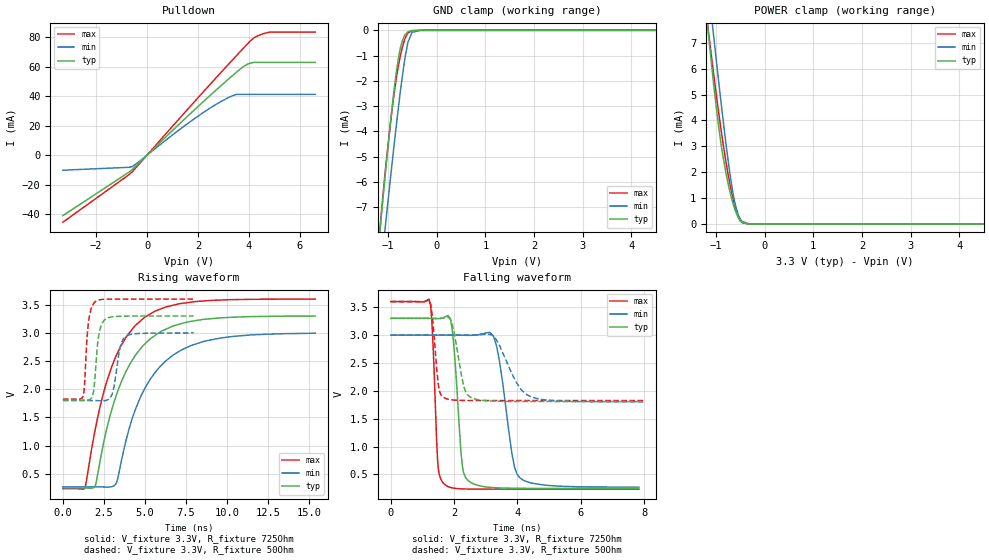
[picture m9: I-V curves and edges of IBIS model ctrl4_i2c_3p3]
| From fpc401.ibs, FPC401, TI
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|   ctrl4_i2c_3p3 Model
[Model]   ctrl4_i2c_3p3
Model_type   I/O_open_drain
Polarity   Non-Inverting
Vinl = 0.8
Vinh = 2
Vmeas = 1.65
Vref = 3.3
Cref = 50pF
Rref = 725
|   typ   min   max
|   (nom PVT)   (fast PVT)   (slow PVT)
C_comp   1.313e-14   1.211e-14   2.018e-14
| Where nom  PVT is Nominal Process, 3.3V, 27C
|   Fast PVT is Strong Process,  3.6V, -40C
|   Slow PVT is Weak Process,   3V, 125C
[Voltage Range]   3.3   3   3.6
|Junction Temperature
[Temperature Range]   27   125   -40
[Pullup Reference]   3.3   3   3.6
[Pulldown Reference]   0   0   0
[Power Clamp Reference]   3.3   3   3.6
[GND Clamp Reference]   0   0   0
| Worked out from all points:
|   slope of the pulldown table from 0 to 0.495 V, typ, clamps not added: 59.6 ohm
|   GND clamp passes 1 mA (typ) near -0.77 V on its own axis
|   POWER clamp passes 1 mA (typ) near -0.68 V on its own axis
|   falling waveform, V_fixture 3.3V, R_fixture 725Ohm: 20-80 % time 216ps typ, 392ps min, 138ps max; typ from 3.3 V to 0.25 V
|   rising waveform, V_fixture 3.3V, R_fixture 725Ohm: 20-80 % time 2.3ns typ, 2.46ns min, 2.13ns max; typ from 0.25 V to 3.3 V
|   falling waveform, V_fixture 3.3V, R_fixture 50Ohm: 20-80 % time 281ps typ, 620ps min, 162ps max; typ from 3.3 V to 1.81 V
|   rising waveform, V_fixture 3.3V, R_fixture 50Ohm: 20-80 % time 290ps typ, 393ps min, 250ps max; typ from 1.81 V to 3.3 V
[Pulldown]
|   Voltage   I(typ)   I(min)   I(max)
-3.3V     -40.84mA   -10.13mA   -45.3mA
-582mV    -9.69mA    -7.733mA   -11.26mA
1.419V    23.6mA     19.21mA    27.73mA
2.042V    33.65mA    26.95mA    39.73mA
2.745V    44.68mA    34.79mA    53.09mA
3.465V    55.55mA    40.96mA    66.6mA
3.792V    60.17mA    41.21mA    72.65mA
3.942V    61.63mA    41.21mA    75.42mA
4.188V    62.83mA    41.21mA    79.35mA
4.469V    62.84mA    41.21mA    81.7mA
4.812V    62.84mA    41.21mA    83.33mA
6.6V      62.84mA    41.21mA    83.34mA
[GND Clamp]
|   Voltage   I(typ)   I(min)   I(max)
-3.3V     -54.89mA   -51.39mA   -65.13mA
-1.185V   -8.379mA   -10.2mA    -8.358mA
-1.136V   -7.374mA   -9.294mA   -7.262mA
-1.063V   -5.874mA   -7.93mA    -5.729mA
-1.036V   -5.337mA   -7.435mA   -5.211mA
-921mV    -3.166mA   -5.372mA   -3.232mA
-813mV    -1.447mA   -3.515mA   -1.711mA
-708mV    -433.5uA   -1.87mA    -696.7uA
-587.4mV  -56.44uA   -464.8uA   -107.3uA
-504mV    -9.281uA   -78.14uA   -15.26uA
-330mV    -89.63nA   -774.9nA   -56.52nA
6.6V      0A         0A         0A
[POWER Clamp]
|   Voltage   I(typ)   I(min)   I(max)
-3.3V     51.03mA    49.04mA    56.86mA
-1.215V   8.494mA    10.26mA    8.507mA
-1.154V   7.358mA    9.183mA    7.481mA
-1.049V   5.476mA    7.341mA    5.852mA
-957mV    3.979mA    5.758mA    4.513mA
-877.8mV  2.896mA    4.444mA    3.437mA
-792mV    1.96mA     3.096mA    2.391mA
-693.6mV  1.114mA    1.72mA     1.378mA
-603.9mV  528.6uA    767.8uA    636.2uA
-537.9mV  234uA      339.3uA    259.2uA
-459.6mV  57.25uA    98.52uA    50.79uA
6.6V      0A         0A         0A
[Ramp]
R_load = 725
|   typ   min   max
dV/dt_r   1.82992/2.30166e-09   1.63827/2.47636e-09   2.01817/2.13245e-09
dV/dt_f   1.82997/2.15714e-10   1.63824/3.92609e-10   2.01826/1.38233e-10
[Falling Waveform]
V_fixture = 3.3V
V_fixture_min = 3V
V_fixture_max = 3.6V
R_fixture = 725Ohm
|   Time   V(typ)   V(min)   V(max)
0s        3.3V       3V         3.6V
1.207ns   3.3V       3V         3.645V
1.501ns   3.294V     3V         601.1mV
1.755ns   3.336V     3V         297.4mV
1.937ns   3.116V     3V         259.7mV
2.263ns   639.5mV    2.997V     241.3mV
2.432ns   397.5mV    2.995V     238.7mV
3.244ns   264.4mV    2.98V      236.3mV
4.074ns   252mV      441.7mV    236.3mV
7.835ns   250.1mV    270.5mV    236.3mV
[Rising Waveform]
V_fixture = 3.3V
V_fixture_min = 3V
V_fixture_max = 3.6V
R_fixture = 725Ohm
|   Time   V(typ)   V(min)   V(max)
0s        250.1mV    269.5mV    236.4mV
1.368ns   249.9mV    269.5mV    271.6mV
1.988ns   298.1mV    270.1mV    1.313V
2.639ns   1.257V     266mV      2.099V
3.244ns   1.881V     325.7mV    2.59V
4.15ns    2.477V     1.409V     3.036V
4.996ns   2.802V     2.015V     3.279V
6.286ns   3.066V     2.506V     3.46V
7.835ns   3.205V     2.779V     3.546V
15.4ns    3.299V     2.994V     3.6V
[Falling Waveform]
V_fixture = 3.3V
V_fixture_min = 3V
V_fixture_max = 3.6V
R_fixture = 50Ohm
|   Time   V(typ)   V(min)   V(max)
0s        3.3V       3V         3.6V
1.207ns   3.3V       3V         3.621V
1.529ns   3.299V     3V         2.013V
1.724ns   3.313V     3V         1.865V
1.94ns    3.196V     3V         1.837V
2.3ns     2.091V     2.999V     1.827V
2.572ns   1.87V      2.999V     1.826V
3.216ns   1.816V     2.994V     1.825V
4.449ns   1.808V     1.887V     1.825V
7.974ns   1.808V     1.801V     1.825V
[Rising Waveform]
V_fixture = 3.3V
V_fixture_min = 3V
V_fixture_max = 3.6V
R_fixture = 50Ohm
|   Time   V(typ)   V(min)   V(max)
0s        1.808V     1.801V     1.825V
1.256ns   1.807V     1.801V     1.905V
1.565ns   1.81V      1.801V     3.194V
1.806ns   1.88V      1.801V     3.488V
1.983ns   2.306V     1.801V     3.555V
2.239ns   3.036V     1.797V     3.587V
2.649ns   3.253V     1.804V     3.598V
3.004ns   3.285V     1.913V     3.6V
3.772ns   3.298V     2.923V     3.6V
7.974ns   3.3V       3V         3.6V
